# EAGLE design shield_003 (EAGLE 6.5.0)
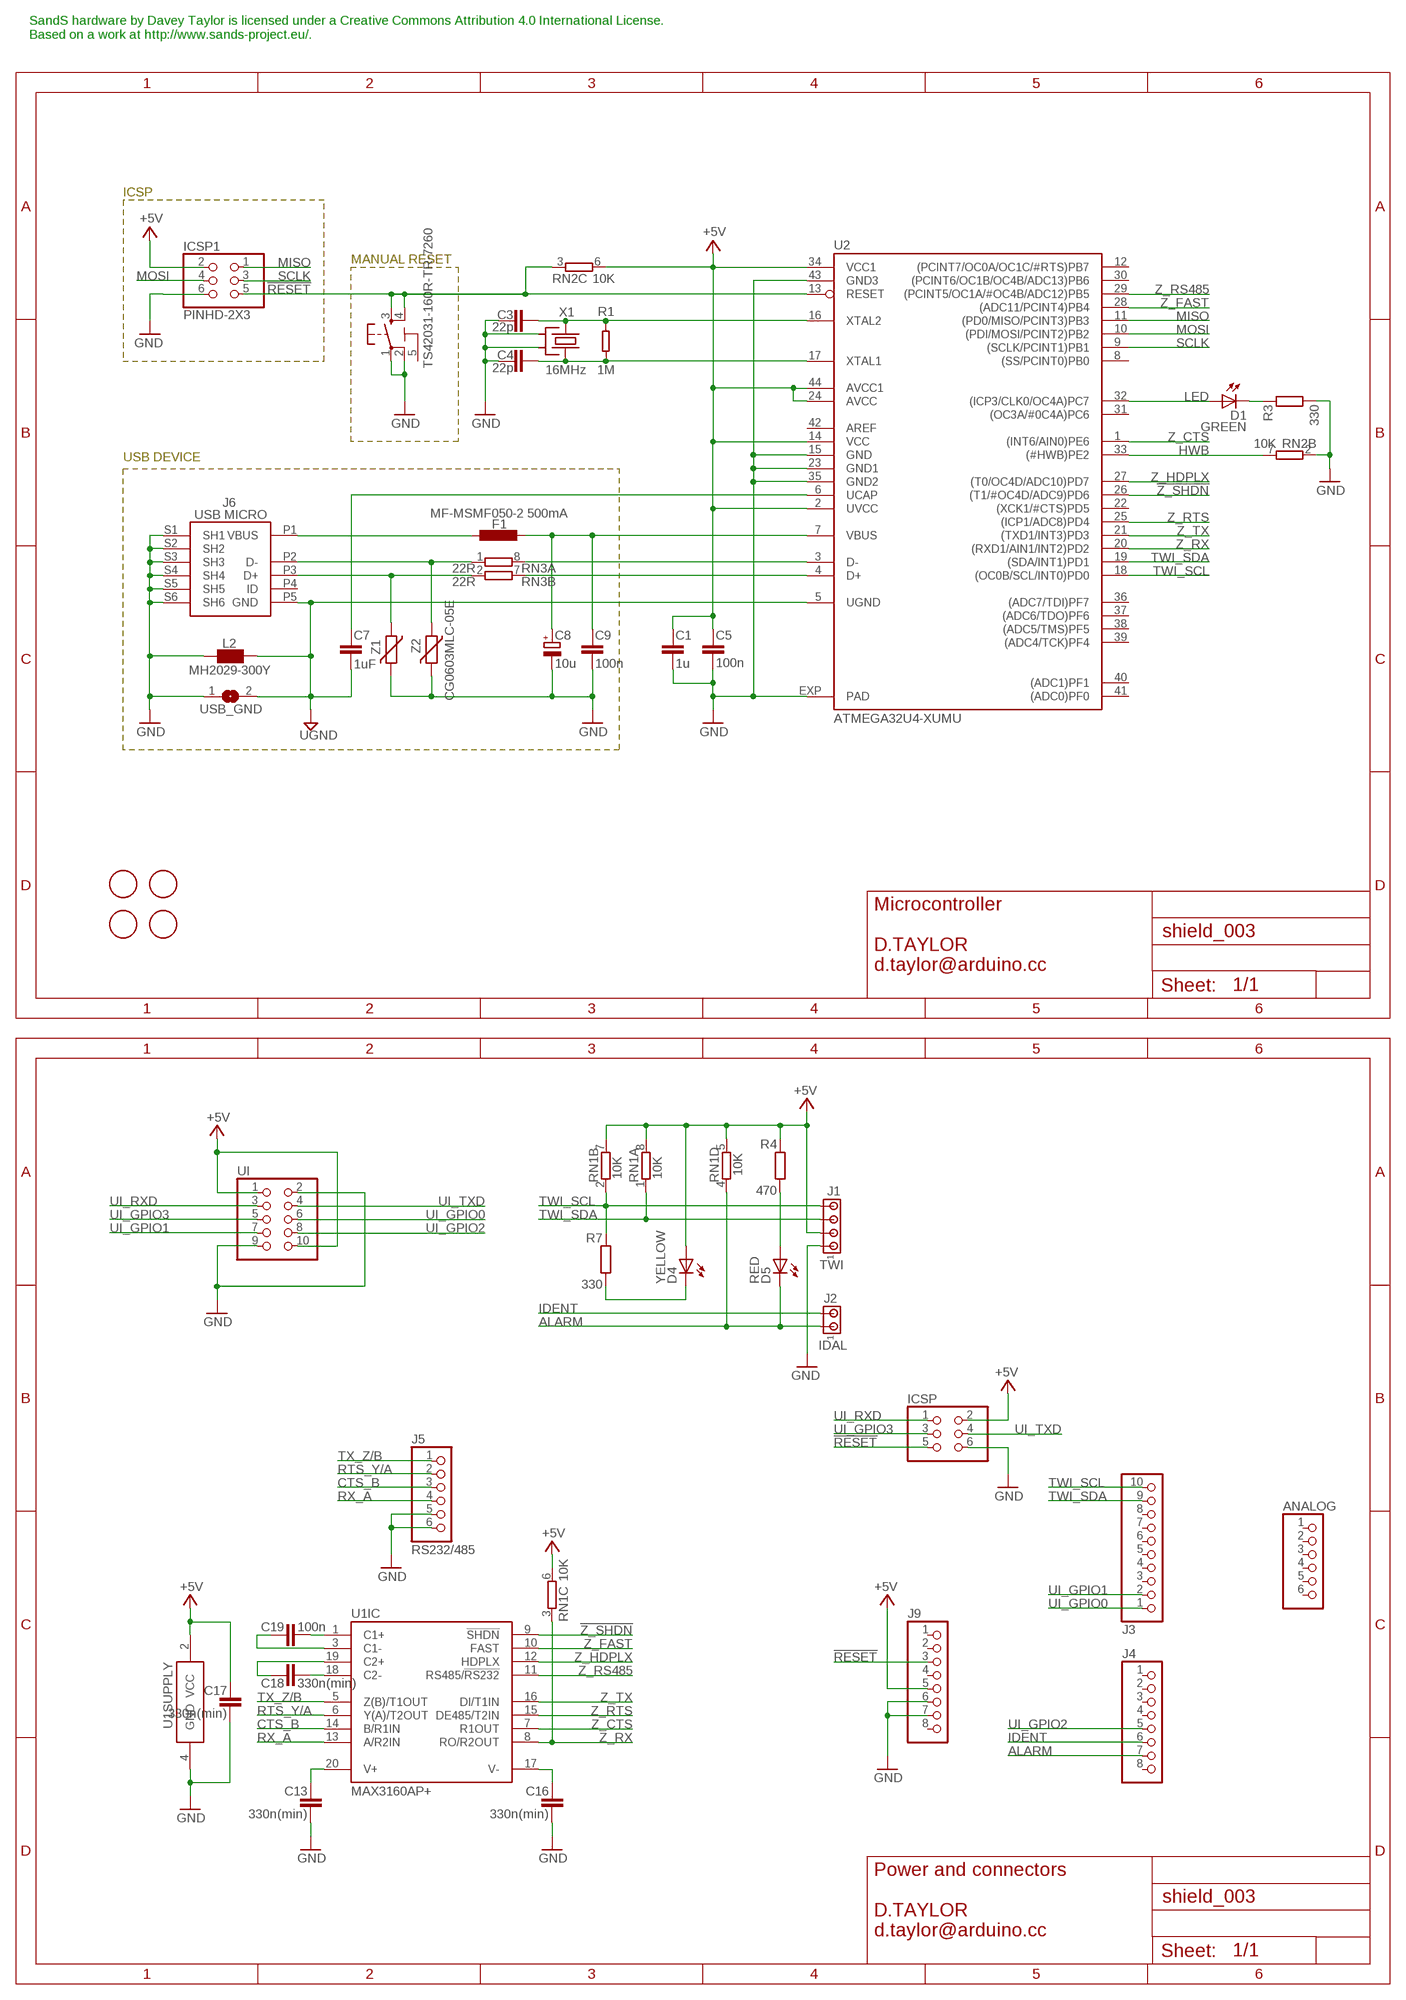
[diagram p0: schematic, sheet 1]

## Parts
ANALOG  PINHD-1X6  [1X06]
C1  1u  C-EUC0603  [C0603-ROUND]
C3  22p  C-EUC0603  [C0603-ROUND]
C4  22p  C-EUC0603  [C0603-ROUND]
C5  100n  C-EUC0603  [C0603-ROUND]
C7  1uF  C-EUC0603  [C0603-ROUND]
C8  10u  CPOL-EUSMCB  [SMC_B]
C9  100n  C-EUC0603  [C0603-ROUND]
C13  330n(min)  C-EU0603-RND  [C0603-ROUND]
C16  330n(min)  C-EU0603-RND  [C0603-ROUND]
C17  330n(min)  C-EU0603-RND  [C0603-ROUND]
C18  330n(min)  C-EU0603-RND  [C0603-ROUND]
C19  100n  C-EU0603-RND  [C0603-ROUND]
D1  GREEN  LEDCHIP-LED0805  [CHIP-LED0805]
D4  YELLOW  LEDCHIP-LED0805  [CHIP-LED0805]
D5  RED  LEDCHIP-LED0805  [CHIP-LED0805]
F1  MF-MSMF050-2 500mA  L-EUL1812  [L1812]
FID1  FIDUCIALMOUNT  [FIDUCIA-MOUNT]
FID2  FIDUCIALMOUNT  [FIDUCIA-MOUNT]
FID4  FIDUCIALMOUNT  [FIDUCIA-MOUNT]
FID5  FIDUCIALMOUNT  [FIDUCIA-MOUNT]
ICSP  PINHD-2X3  [2X03]
ICSP1  PINHD-2X3  [2X03]
J1  TWI  MTA04-100  [10X04MTA]
J2  IDAL  MTA02-100  [10X02MTA]
J3  PINHD-1X10TH  [1X10-TH]
J4  PINHD-1X8TH  [1X08-TH]
J5  RS232/485  PINHD-1X6  [1X06]
J6  USB MICRO  MYCON2_USB-MINI-B  [CON2_USB_MICRO_B_AT]
J9  PINHD-1X8TH  [1X08-TH]
L2  MH2029-300Y  WE-CBF_0805  [0805]
R1  1M  R-EU_0603-RND  [R0603-ROUND]
R3  330  R-EU_R0603  [R0603-ROUND]
R4  470  R-EU_R0603  [R0603-ROUND]
R7  330  R-EU_R0603  [R0603-ROUND]
RESET1  TS42031-160R-TR-7260  TS42  [TS42]
RN1  10K  4R-NCAT16  [CAT16]
RN2  10K  4R-NCAY16  [CAY16]
RN3  22R  4R-NCAY16  [CAY16]
U1  MAX3160AP+  [SSOP20]
U2  ATMEGA32U4-XUMU  [QFN44ML7X7]
UI  PINHD-2X5  [2X05]
USB_GND  SJ-NO  [SJ]
X1  16MHz  CRYSTAL2-KX7  [XTAL-3.2-2.5]
Z1  CG0603MLC-05E  VARISTORCN0603  [CT/CN0603]
Z2  CG0603MLC-05E  VARISTORCN0603  [CT/CN0603]

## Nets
!RESET!: ICSP1.5 ICSP.5 J9.3 RESET1.3 RESET1.4 RN2.3 U2.13(RESET)
!Z_SHDN!: U1.9(IC:!SHDN!) U2.26((T1/#OC4D/ADC9)PD6)
+5V: C1.1 C5.1 C17.1 D4.A ICSP1.2 ICSP.2 J1.2 J9.5 R4.2 RN1.5 RN1.6 RN1.7 RN1.8 RN2.6 U1.2(SUPPLY:VCC) U2.2(UVCC) U2.14(VCC) U2.24(AVCC) U2.34(VCC1) U2.44(AVCC1) UI.1 UI.10
ALARM: D5.C J2.1 J4.7 RN1.4
CTS_B: J5.3 U1.14(IC:B/R1IN)
D+: J6.P3(D+) RN3.2 Z1.1
D-: J6.P2(D-) RN3.1 Z2.1
GND: C1.2 C3.1 C4.2 C5.2 C8.- C9.2 C13.2 C16.2 C17.2 ICSP1.6 ICSP.6 J1.1 J5.5 J5.6 J6.S1(SH1) J6.S2(SH2) J6.S3(SH3) J6.S4(SH4) J6.S5(SH5) J6.S6(SH6) J9.6 J9.7 L2.2 R3.1 RESET1.1 RESET1.2 RN2.2 U1.4(SUPPLY:GND) U2.15(GND) U2.23(GND1) U2.35(GND2) U2.43(GND3) U2.EXP(PAD) UI.2 UI.9 USB_GND.1 X1.2(SH1) X1.4(SH2) Z1.2 Z2.2
HWB: RN2.7 U2.33((#HWB)PE2)
IDENT: J2.2 J4.6
LED: D1.A U2.32((ICP3/CLK0/OC4A)PC7)
MISO: ICSP1.1 U2.11((PD0/MISO/PCINT3)PB3)
MOSI: ICSP1.4 U2.10((PDI/MOSI/PCINT2)PB2)
N$2: D1.C R3.2
N$5: D5.A R4.1
N$6: C19.2 U1.1(IC:C1+)
N$7: C18.2 U1.18(IC:C2-)
N$8: C18.1 U1.19(IC:C2+)
N$9: C19.1 U1.3(IC:C1-)
N$10: C13.1 U1.20(IC:V+)
N$11: C16.1 U1.17(IC:V-)
N$14: D4.C R7.1
RTS_Y/A: J5.2 U1.6(IC:Y(A)/T2OUT)
RX_A: J5.4 U1.13(IC:A/R2IN)
SCLK: ICSP1.3 U2.9((SCLK/PCINT1)PB1)
TWI_SCL: J1.4 J3.10 R7.2 RN1.2 U2.18((OC0B/SCL/INT0)PD0)
TWI_SDA: J1.3 J3.9 RN1.1 U2.19((SDA/INT1)PD1)
TX_Z/B: J5.1 U1.5(IC:Z(B)/T1OUT)
UCAP: C7.1 U2.6(UCAP)
UGND: C7.2 J6.P5(GND) L2.1 U2.5(UGND) USB_GND.2
UI_GPIO0: J3.1 UI.6
UI_GPIO1: J3.2 UI.7
UI_GPIO2: J4.5 UI.8
UI_GPIO3: ICSP.3 UI.5
UI_RXD: ICSP.1 UI.3
UI_TXD: ICSP.4 UI.4
USB_D+: RN3.7 U2.4(D+)
USB_D-: RN3.8 U2.3(D-)
USB_VCC: C8.+ C9.1 F1.1 U2.7(VBUS)
XTAL1: C4.1 R1.1 U2.17(XTAL1) X1.3(X2)
XTAL2: C3.2 R1.2 U2.16(XTAL2) X1.1(X1)
XUSB [power usb]: F1.2 J6.P1(VBUS)
Z_CTS: U1.7(IC:R1OUT) U2.1((INT6/AIN0)PE6)
Z_FAST: U1.10(IC:FAST) U2.28((ADC11/PCINT4)PB4)
Z_HDPLX: U1.12(IC:HDPLX) U2.27((T0/OC4D/ADC10)PD7)
Z_RS485: U1.11(IC:RS485/!RS232!) U2.29((PCINT5/OC1A/#OC4B/ADC12)PB5)
Z_RTS: U1.15(IC:DE485/T2IN) U2.25((ICP1/ADC8)PD4)
Z_RX: RN1.3 U1.8(IC:RO/R2OUT) U2.20((RXD1/AIN1/INT2)PD2)
Z_TX: U1.16(IC:DI/T1IN) U2.21((TXD1/INT3)PD3)
Unconnected: ANALOG.1 ANALOG.2 ANALOG.3 ANALOG.4 ANALOG.5 ANALOG.6 J3.3 J3.4 J3.5 J3.6 J3.7 J3.8 J4.1 J4.2 J4.3 J4.4 J4.8 J6.P4(ID) J9.1 J9.2 J9.4 J9.8 RN2.1 RN2.4 RN2.5 RN2.8 RN3.3 RN3.4 RN3.5 RN3.6 U2.8((SS/PCINT0)PB0) U2.12((PCINT7/OC0A/OC1C/#RTS)PB7) U2.22((XCK1/#CTS)PD5) U2.30((PCINT6/OC1B/OC4B/ADC13)PB6) U2.31((OC3A/#0C4A)PC6) U2.36((ADC7/TDI)PF7) U2.37((ADC6/TDO)PF6) U2.38((ADC5/TMS)PF5) U2.39((ADC4/TCK)PF4) U2.40((ADC1)PF1) U2.41((ADC0)PF0)

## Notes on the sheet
- SandS hardware by Davey Taylor is licensed under a Creative Commons Attribution 4.0 International License.
  Based on a work at http://www.sands-project.eu/.
- ICSP
- MANUAL RESET
- USB DEVICE
- Microcontroller
  
  D.TAYLOR
  d.taylor@arduino.cc
- Power and connectors
  
  D.TAYLOR
  d.taylor@arduino.cc

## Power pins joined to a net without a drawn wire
5-GND: RESET1.5(5-GND)
AREF: U2.42(AREF)

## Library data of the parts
ANALOG J5 = pinhead:PINHD-1X6: PIN HEADER
C1 C3-C5 C7 C9 C13 C16-C19 = SmartPrj:C-EU: CAPACITOR, European symbol
C8 = rcl:CPOL-EU: POLARIZED CAPACITOR, European symbol
D1 D4 D5 = led:LED: LED
F1 = rcl:L-EU: INDUCTOR, European symbol
FID1 FID2 FID4 FID5 = SmartPrj:FIDUCIALMOUNT
ICSP ICSP1 = SmartPrj:PINHD-2X3: PIN HEADER
J1 = con-amp:MTA04-100: AMP connector
J2 = con-amp:MTA02-100: AMP connector
J3 = SmartPrj:PINHD-1X10: PIN HEADER
J4 J9 = SmartPrj:PINHD-1X8: PIN HEADER
J6 = d_taylor:MYCON2_USB-MINI-B
L2 = wuerth-elektronik:WE-CBF: SMD EMI Suppression Ferrite Beads
R1 = d_taylor:R-EU_: RESISTOR, European symbol
R3 R4 R7 = SmartPrj:R-EU_: RESISTOR, European symbol
RESET1 = SmartPrj:TS42: TS42 Dongnan Electronics Tact switch VDC 12V - 50mA
RN1-RN3 = resistor-dil:4R-N: Array Chip Resistor Source: RS Component / Phycomp; OC_FARNELL: unknown; OC_NEWARK: unknown
U1 = d_taylor:MAX3160*AP+
U2 = d_taylor:ATMEGA32U4-XU
UI = pinhead:PINHD-2X5: PIN HEADER
USB_GND = d_taylor:SJ?-NO: SMD solder JUMPER
X1 = d_taylor:CRYSTAL2: KX7 SMD crystal
Z1 Z2 = varistor:VARISTOR: VARISTOR

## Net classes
0 default: width 0.203 mm, drill 0.406 mm, clearance 0.203 mm
1 power: width 0.61 mm, drill 0.406 mm, clearance 0.203 mm
2 gnd: width 0.305 mm, drill 0.406 mm, clearance 0.203 mm
3 power usb: width 0.508 mm, drill 0.406 mm, clearance 0.203 mm
4 aref: width 0.203 mm, drill 0.406 mm, clearance 0.203 mm

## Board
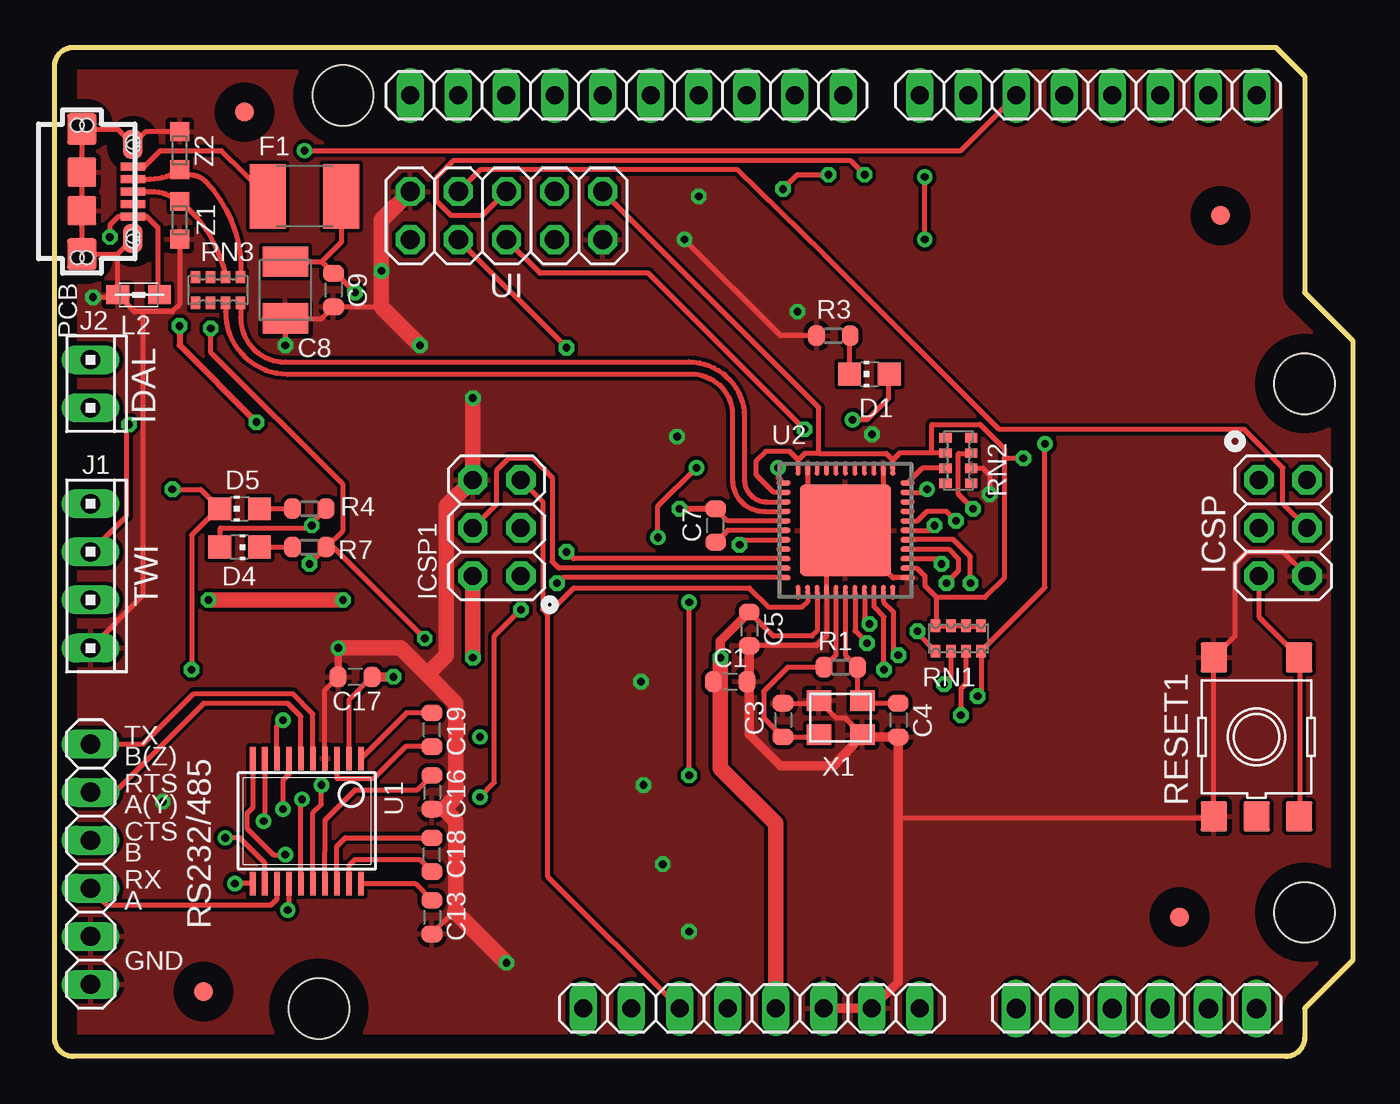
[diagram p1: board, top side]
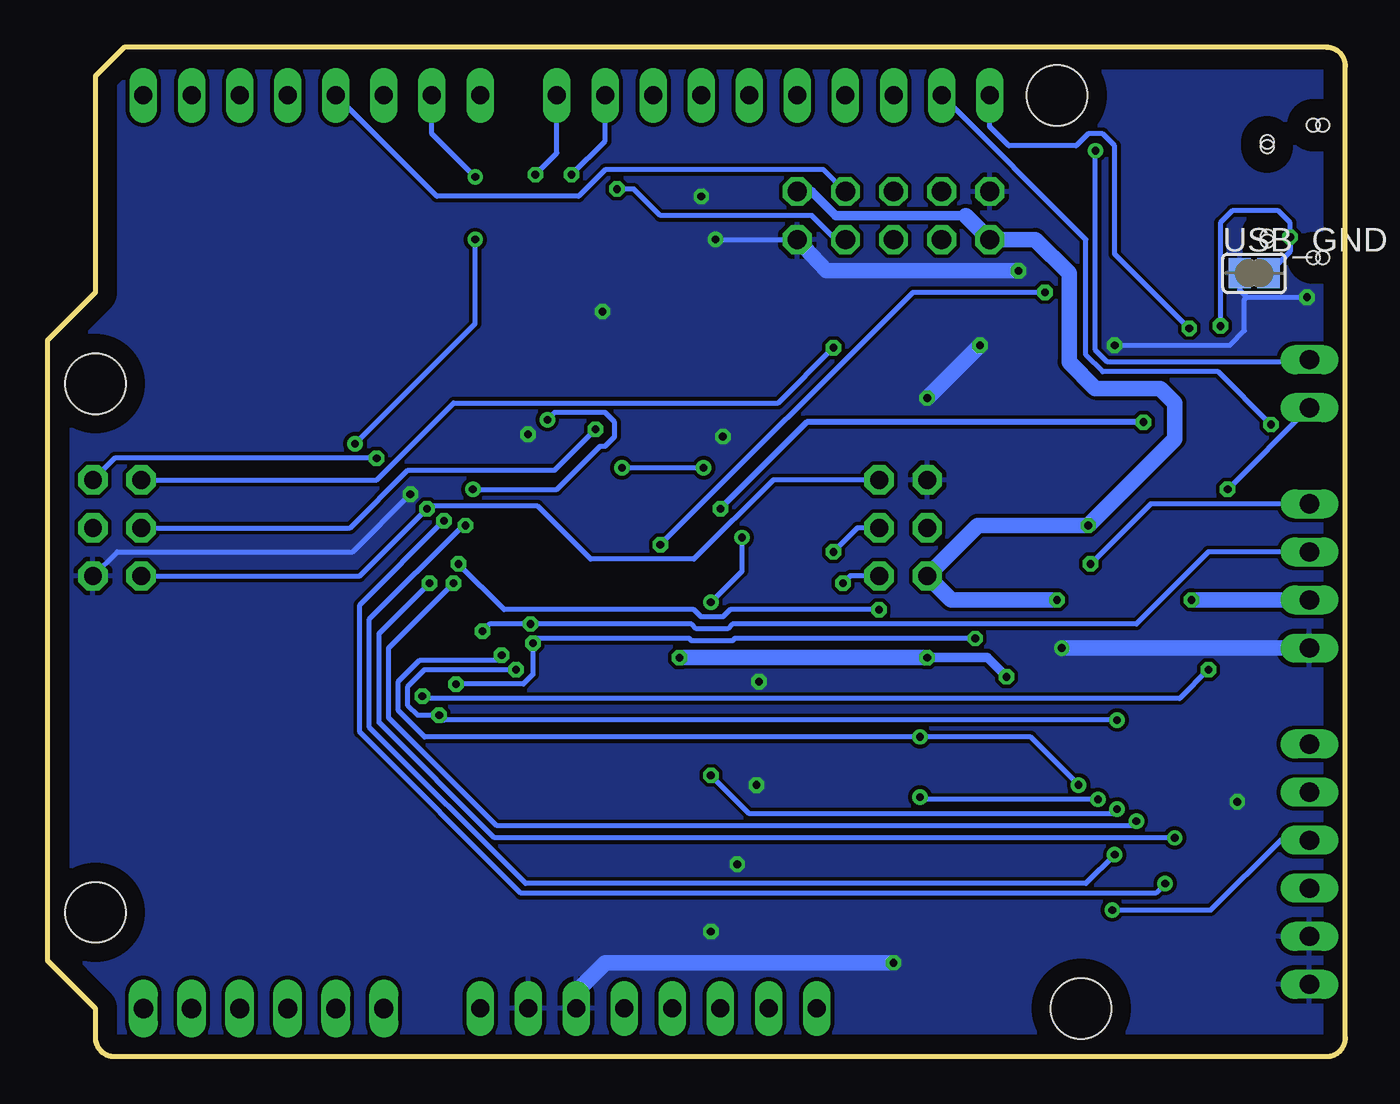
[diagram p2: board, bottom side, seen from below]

Size 68.58 x 53.34 mm. Coordinates in mm from the lower left corner, seen from the top.
Outline: 64.52,53.34 66.04,51.82 66.04,40.39 68.58,37.85 68.58,5.08 66.04,2.54 66.04,1 arc-90 65.04,0 1,0 arc-90 0,1 0,52.34 arc-90 1,53.34 64.52,53.34
Copper layers (1*16): Top 0.035mm / dielectric 1.5mm / Bottom 0.035mm
Design rules "default *": minimum track width 10mil, minimum drill 16mil, track to track 8mil, track to pad 8mil, pad to pad 8mil, via to via 8mil, smd to smd 8mil, copper to edge 40mil, drill to drill 8mil, minimum pad ring 10mil, minimum via ring 8mil, stop-mask expansion 4mil, vias tented up to drill 0mil, thermal gap 10mil
Holes 3.2 mm at 66.04,35.56 66.04,7.62 15.24,50.8 13.97,2.54

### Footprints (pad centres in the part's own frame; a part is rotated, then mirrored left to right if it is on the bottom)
1X06 = drill 1.016 long: 1 -6.35,0; 2 -3.81,0; 3 -1.27,0; 4 1.27,0; 5 3.81,0; 6 6.35,0
C0603-ROUND = smd 0.898 x 1.1: 1 -0.889,0; 2 0.889,0
SMC_B = smd 1.6 x 2.4: + -1.5,0; - 1.5,0
CHIP-LED0805 = smd 1.2 x 1.2: A 0,-1.05; C 0,1.05
L1812 = smd 1.9 x 3.4: 1 -1.95,0; 2 1.95,0
FIDUCIA-MOUNT = smd 1.016 x 1.016: P$1 0,0
2X03 = drill 0.95 pad 1.55 octagon: 1 -2.54,-1.27; 2 -2.54,1.27; 3 0,-1.27; 4 0,1.27; 5 2.54,-1.27; 6 2.54,1.27
10X04MTA = drill 1.016 long: 1 3.81,0; 2 1.27,0; 3 -1.27,0; 4 -3.81,0
10X02MTA = drill 1.016 long: 1 1.27,0; 2 -1.27,0
1X10-TH = drill 0.95 pad 1.422 long: 1 -11.43,0; 2 -8.89,0; 3 -6.35,0; 4 -3.81,0; 5 -1.27,0; 6 1.27,0; 7 3.81,0; 8 6.35,0; 9 8.89,0; 10 11.43,0
1X08-TH = drill 0.95 pad 1.422 long: 1 -8.89,0; 2 -6.35,0; 3 -3.81,0; 4 -1.27,0; 5 1.27,0; 6 3.81,0; 7 6.35,0; 8 8.89,0
CON2_USB_MICRO_B_AT = smd 0.406 x 1.346: P1 -1.321,2.692; P2 -0.66,2.692; P3 0,2.692; P4 0.66,2.692; P5 1.321,2.692 | smd 1.651 x 1.549: S1 -3.302,0; S2 3.302,0 | smd 1.524 x 1.016: S3 -2.489,2.692; S4 2.489,2.692 | smd 1.524 x 1.524: S5 -1.016,0; S6 1.016,0 | hole 0.7: -3.505,0.254; -3.505,-0.254; 3.505,0.254; 3.505,-0.254; -2.616,2.692; -2.362,2.692; 2.362,2.692; 2.616,2.692
0805 = smd 1.2 x 1: 1 -1.1,0; 2 1.1,0
R0603-ROUND = smd 0.898 x 1.1: 1 -0.889,0; 2 0.889,0
TS42 = smd 1.6 x 1.4: 1 -4.2,2.25; 2 4.2,2.25; 3 -4.2,-2.25; 4 4.2,-2.25; 5 -4.2,0
CAT16 = smd 0.5 x 0.65: 1 -1.2,-0.675; 2 -0.4,-0.675; 3 0.4,-0.675; 4 1.2,-0.675; 5 1.2,0.675; 6 0.4,0.675; 7 -0.4,0.675; 8 -1.2,0.675
CAY16 = smd 0.5 x 0.65: 1 -1.2,-0.675; 2 -0.4,-0.675; 3 0.4,-0.675; 4 1.2,-0.675; 5 1.2,0.675; 6 0.4,0.675; 7 -0.4,0.675; 8 -1.2,0.675
SSOP20 = smd 0.305 x 1.245: 1 -2.857,-3.302; 2 -2.222,-3.302; 3 -1.587,-3.302; 4 -0.952,-3.302; 5 -0.317,-3.302; 6 0.318,-3.302; 7 0.953,-3.302; 8 1.588,-3.302; 9 2.223,-3.302; 10 2.858,-3.302; 11 2.858,3.302; 12 2.223,3.302; 13 1.588,3.302; 14 0.953,3.302; 15 0.318,3.302; 16 -0.317,3.302; 17 -0.952,3.302; 18 -1.587,3.302; 19 -2.222,3.302; 20 -2.857,3.302
QFN44ML7X7 = smd 0.75 x 0.275: 1 -3.275,2.5; 2 -3.275,2; 3 -3.275,1.5; 4 -3.275,1; 5 -3.275,0.5; 6 -3.275,0; 7 -3.275,-0.5; 8 -3.275,-1; 9 -3.275,-1.5; 10 -3.275,-2; 11 -3.275,-2.5; 23 3.275,-2.5; 24 3.275,-2; 25 3.275,-1.5; 26 3.275,-1; 27 3.275,-0.5; 28 3.275,0; 29 3.275,0.5; 30 3.275,1; 31 3.275,1.5; 32 3.275,2; 33 3.275,2.5 | smd 0.275 x 0.75: 12 -2.5,-3.275; 13 -2,-3.275; 14 -1.5,-3.275; 15 -1,-3.275; 16 -0.5,-3.275; 17 0,-3.275; 18 0.5,-3.275; 19 1,-3.275; 20 1.5,-3.275; 21 2,-3.275; 22 2.5,-3.275; 34 2.5,3.275; 35 2,3.275; 36 1.5,3.275; 37 1,3.275; 38 0.5,3.275; 39 0,3.275; 40 -0.5,3.275; 41 -1,3.275; 42 -1.5,3.275; 43 -2,3.275; 44 -2.5,3.275 | smd 4.826 x 4.826: EXP 0,0
2X05 = drill 1.016 octagon: 1 -5.08,-1.27; 2 -5.08,1.27; 3 -2.54,-1.27; 4 -2.54,1.27; 5 0,-1.27; 6 0,1.27; 7 2.54,-1.27; 8 2.54,1.27; 9 5.08,-1.27; 10 5.08,1.27
SJ = smd 1.168 x 1.6: 1 -0.762,0; 2 0.762,0
XTAL-3.2-2.5 = smd 1.3 x 1.1: 1 -1.15,-0.9; 2 1.15,-0.9; 3 1.15,0.9; 4 -1.15,0.9
CT/CN0603 = smd 1 x 1: 1 -1,0; 2 1,0

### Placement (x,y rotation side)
ANALOG  57.15,2.54 0 top
C1  35.69,19.81 0 top
C3  38.48,17.78 270 top
C4  44.58,17.78 270 top
C5  36.7,22.61 270 top
C7  34.92,28.07 90 top
C8  12.19,40.51 270 top
C9  14.73,40.51 270 top
C13  19.94,7.37 270 top
C16  19.94,13.97 270 top
C17  15.88,20.07 180 top
C18  19.94,10.67 90 top
C19  19.94,17.27 90 top
D1  43.05,36.07 90 top
D4  9.78,26.92 270 top
D5  9.78,28.96 90 top
F1  13.21,45.47 180 top
FID1  10.03,49.91 0 top
FID2  7.87,3.43 0 top
FID4  61.59,44.45 0 top
FID5  59.44,7.37 0 top
ICSP  64.9,27.94 270 top
ICSP1  23.37,27.94 90 top
J1  1.91,25.4 270 top
J2  1.91,35.56 270 top
J3  30.23,50.8 180 top
J4  54.61,50.8 180 top
J5  1.91,10.16 270 top
J6  1.45,45.72 270 top
J9  36.83,2.54 0 top
L2  4.45,40.26 180 top
R1  41.53,20.57 180 top
R3  41.15,38.1 0 top
R4  13.46,28.96 0 top
R7  13.46,26.92 0 top
RESET1  63.5,16.89 90 top
RN1  47.75,22.1 0 top
RN2  47.75,31.5 90 top
RN3  8.64,40.51 180 top
U1  13.34,12.45 180 top
U2  41.78,27.81 0 top
UI  23.88,44.45 0 top
USB_GND  4.83,41.4 0 bottom
X1  41.53,17.91 0 top
Z1  6.6,44.2 270 top
Z2  6.6,47.88 90 top

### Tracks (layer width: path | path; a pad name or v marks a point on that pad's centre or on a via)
!RESET!  (via drill 0.41)
  Top 0.254: RESET1.3 65.79,12.7 65.79,21.08 RESET1.4 65.66,21.21 63.63,23.24 ICSP.5 | v48.51,28.96 47.75,29.72 47.75,31.88 48.26,31.88 RN2.3 | 26.04,23.37 27.43,24.77 36.7,24.77 37.72,23.75 39.5,23.75 39.78,24.04 U2.13 | 26.04,23.37 25.78,23.62 25.78,29.34 ICSP1.5 | J9.3 26.04,9.53 26.04,23.37
  Bottom 0.254: ICSP.5 52.07,25.4 v48.51,28.96 48.39,29.08 42.67,29.08 39.88,26.29 34.42,26.29 30.23,30.48 ICSP1.5
!Z_SHDN!  (via drill 0.41)
  Top 0.254: v47.12,25.02 47.74,25.67 47.75,25.69 47.75,26.29 47.23,26.81 U2.26 | U1.9 11.11,12.51 v11.05,12.45
  Bottom 0.254: v47.12,25.02 50.55,21.59 50.55,17.91 44.83,12.19 11.3,12.19 v11.05,12.45
+5V  (via drill 0.41)
  Top 0.254: 16.75,20.05 C17.1 15.56,18.86 U1.2 | RN2.6 46.35,31.9 | U2.14 40.28,22.5 40.01,22.23 37.97,22.23 C5.1 36.83,23.24 | 13.53,28.13 13.34,27.94 8.76,27.94 8.76,26.92 D4.A 8.64,26.92 | 13.53,28.13 R4.2 | v13.59,28.07 13.53,28.13 | RN1.5 48.9,22.73 48.26,22.73 RN1.6 RN1.7 47.24,22.73 46.61,22.73 RN1.8 46.61,22.86 46.61,24.26 | 40.39,31.88 39.62,31.88 39.28,31.54 | 46.61,24.26 49.15,24.26 50.16,25.27 50.16,31.62 | 50.16,31.62 50.16,32.13 48.9,33.4 46.35,33.4 46.35,31.9 | 50.16,31.62 v51.18,31.62 | UI.10 40.39,34.29 40.39,31.88 | 40.39,31.88 43.94,31.88 44.28,31.54 | 46.35,31.9 44.64,31.9 44.28,31.54 | U2.34 44.28,31.54 | U2.44 39.28,31.54 | U2.2 38.01,29.81 37.08,30.73 37.08,31.5 37.56,31.98 38.84,31.98 39.28,31.54 | U2.24 45.56,25.81 45.97,25.4 45.97,24.89 46.61,24.26
  Top 0.406: C1.1 35.18,19.81
  Top 0.508: v17.91,20.07 C17.1 | v35.18,21.08 35.18,21.97 C5.1
  Top 0.813: ICSP1.2 v22.1,21.08 | J9.5 38.1,12.32 35.18,15.24 35.18,19.81 v35.18,21.08 | v8.13,24.13 v15.24,24.13
  Bottom 0.254: ICSP.2 65.02,31.62 v51.18,31.62
  Bottom 0.508: v17.91,20.07 18.92,21.08 v22.1,21.08 | 20.07,44.45 26.92,44.45 28.19,45.72 UI.10
  Bottom 0.813: v8.13,24.13 J1.2 | v22.1,21.08 v35.18,21.08 | 20.07,44.45 UI.1 16.38,43.18 14.61,41.4 14.61,36.7 13.21,35.31 9.78,35.31 9.02,34.54 9.02,32.64 v13.59,28.07 19.43,28.07 ICSP1.2 20.83,24.13 v15.24,24.13
ALARM  (via drill 0.41)
  Top 0.254: v7.24,20.45 7.24,27.56 8.64,28.96 D5.C 7.71,29.97 v6.22,29.97 | 48.9,21.34 RN1.4 | RN1.4 48.95,19.23 v48.77,19.05 | RN1.4 52.32,24.8 v52.32,32.38 | v45.97,43.18 v45.97,46.48
  Bottom 0.254: v48.77,19.05 48.64,18.92 8.76,18.92 v7.24,20.45 | v6.22,29.97 J2.1 | v52.32,32.38 45.97,38.73 v45.97,43.18 | v45.97,46.48 48.26,48.77 J4.7
CTS_B  (via drill 0.41)
  Top 0.254: U1.14 12.38,7.94 v12.32,7.75
  Bottom 0.254: v12.32,7.75 7.11,7.75 3.43,11.43 J5.3
D+
  Top 0.254: J6.P3 5.08,45.72 arc-38 Z1.1 arc-42 RN3.2
D-
  Top 0.254: J6.P2 5.08,46.38 arc36 Z2.1 6.6,46.61 7.11,46.61 arc-46 8,46.23 arc-47 RN3.1
GND  (via drill 0.41)
  Top 0.254: 14.8,19.88 C17.2 14.29,19.37 U1.4 | 21.21,7.75 21.14,7.68 C13.2 | 3.33,42.42 J6.S2 J6.S6 J6.S5 J6.S1 3.33,49.02 J6.S3 4.81,48.88 Z2.2 | 3.33,42.42 J6.S4 4.19,43.18 | L2.2 3.35,42.4 3.33,42.42 | v2.03,40.13 3.22,40.13 L2.2 | Z1.2 6.6,39.75 6.22,39.37 4.7,39.37 | 4.7,39.37 4.23,39.37 L2.2 | v12.19,37.59 C8.- 14.12,39.01 C9.2 17.27,39.62 | U2.43 39.78,29.81 U2.EXP | U2.35 43.78,29.81 U2.EXP | U2.23 44.28,25.31 U2.EXP | U2.EXP 40.78,26.81 U2.15 40.78,22.24 40.26,21.72 C5.2 | C3.1 40.24,18.67 X1.4 41.28,17.91 41.78,17.91 X1.2 | 4.7,39.37 4.7,24.38 J1.1 | 61.21,12.7 61.21,21.08 RESET1.2 61.34,21.21 62.36,22.23 62.36,26.04 62.99,26.67 64.9,26.67 ICSP.6 | 61.21,12.7 61.21,12.57 44.58,12.57 | 61.21,12.7 RESET1.1 | RN2.2 49.04,31.1 49.4,30.73 v49.4,29.72 | R3.1 38.35,38.1 v33.27,43.18
  Top 0.406: v14.99,21.59 C17.2 | C1.2 36.7,19.81
  Top 0.508: 42.8,16.89 C4.2 44.58,12.57 44.58,3.94 J9.7 J9.6 | C5.2 36.7,19.81 36.7,17.02 38.35,15.37 41.17,15.37 X1.2
  Top 0.813: 20.57,13.08 21.21,12.45 21.21,7.75 | C16.2 20.57,13.08 | 20.57,13.08 21.21,13.72 21.21,18.67 19.68,20.19 | 19.68,20.19 18.29,21.59 v14.99,21.59 | UI.2 17.27,44.2 v17.27,41.53 17.27,39.62 v19.3,37.59 | v23.88,4.95 21.14,7.68 | 19.68,20.19 20.7,21.21 20.7,29.08 ICSP1.6 v22.1,34.8
  Bottom 0.254: USB_GND.1 5.59,40.51 5.21,40.13 | 5.21,40.13 v2.03,40.13 | v12.19,37.59 6.1,37.59 5.33,38.35 5.33,40.01 5.21,40.13 | v49.4,29.72 52.45,26.67 64.9,26.67 ICSP.6 | v33.27,43.18 UI.9
  Bottom 0.813: UI.9 27.43,41.53 v17.27,41.53 | v14.99,21.59 J1.1 | v23.88,4.95 39.12,4.95 40.64,3.43 J9.6 | v22.1,34.8 v19.3,37.59
  other vias: 39.24,39.37 34.04,45.47 32.89,32.77 33.53,6.6 31.11,14.35 43.18,32.89 5.71,13.46 30.99,19.81 32.13,10.16
  pour Bottom: 0.89,0.89 65.15,0.89 65.15,2.79 67.69,5.33 67.69,37.59 65.15,40.13 65.15,52.58 0.89,52.58
  pour Top: 0.89,0.89 65.15,0.89 65.15,2.79 67.69,5.33 67.69,37.59 65.15,40.13 65.15,52.58 0.89,52.58
HWB
  Top 0.254: RN2.7 45.84,31.1 U2.33
IDENT  (via drill 0.41)
  Top 0.254: v13.21,47.88 47.88,47.88 J4.6
  Bottom 0.254: J2.2 2.03,36.7 12.57,36.7 13.21,37.34 v13.21,47.88
LED  (via drill 0.41)
  Top 0.254: U2.32 45.94,29.81 v46.1,29.97 | v42.16,33.66 42.93,33.66 44.07,34.8 44.07,36.03 D1.A
  Bottom 0.254: v46.1,29.97 41.66,29.97 39.37,32.26 39.12,32.26 38.61,32.77 38.61,33.53 39.12,34.04 41.78,34.04 v42.16,33.66
MISO  (via drill 0.41)
  Top 0.254: U2.11 26.84,25.31 v26.54,25.02
  Bottom 0.254: v26.54,25.02 26.16,25.4 ICSP1.1
MOSI
  Top 0.254: ICSP1.4 23.37,29.21 23.37,30.99 24,31.62 25.27,31.62 26.29,30.61 26.29,26.16 26.64,25.81 U2.10
N$2
  Top 0.254: D1.C 42,38.07 R3.2
N$5
  Top 0.254: D5.A R4.1
N$6
  Top 0.254: C19.2 18.61,18.16 U1.1
N$7
  Top 0.254: U1.18 14.92,11.11 15.37,11.56 C18.2
N$8
  Top 0.254: U1.19 15.56,10.1 15.88,10.41 19.3,10.41 C18.1
N$9
  Top 0.254: C19.1 18.54,16.38 16.86,14.7 14.92,14.7 U1.3
N$10
  Top 0.254: U1.20 19.05,9.14 C13.1
N$11
  Top 0.254: U1.17 14.29,12.51 15.88,14.1 19.18,14.1 C16.1
N$14
  Top 0.254: D4.C R7.1
RTS_Y/A
  Top 0.254: J5.2 3.17,13.97 7.87,18.67 12.32,18.67 13.02,17.97 U1.6
RX_A
  Top 0.254: U1.13 11.75,8.32 11.43,8 2.79,8 J5.4
SCLK  (via drill 0.41)
  Top 0.254: U2.9 27.41,26.31 v27.05,26.67
  Bottom 0.254: v27.05,26.67 25.78,27.94 ICSP1.3
TWI_SCL  (via drill 0.41)
  Top 0.254: v13.46,26.04 R7.2 | v8.26,38.48 8.26,37.21 15.24,30.23 15.24,27.81 R7.2 | v42.93,21.84 42.29,22.48 42.29,24.51 U2.18 | RN1.2 47.35,20.05 v46.99,19.68 | R7.2 14.73,26.92 v19.56,22.1
  Bottom 0.254: v46.99,19.68 43.43,19.68 42.93,20.19 v42.93,21.84 42.67,22.1 34.67,22.1 34.54,21.97 32.38,21.97 32.26,22.1 v19.56,22.1 | v13.46,26.04 10.29,29.21 J1.4 | J3.10 18.8,49.15 17.78,48.13 14.22,48.13 13.59,48.77 12.83,48.77 12.19,48.13 12.19,42.42 v8.26,38.48
TWI_SDA  (via drill 0.41)
  Top 0.254: v45.59,22.48 45.59,22.35 46.48,21.46 RN1.1 | U2.19 42.8,24.51 42.8,23.11 v43.05,22.86 | v3.94,33.4 3.81,33.27 3.81,28.57 J1.3
  Bottom 0.254: v45.59,22.48 45.21,22.86 v43.05,22.86 34.54,22.86 34.29,22.61 32.64,22.61 32.38,22.86 11.05,22.86 7.24,26.67 J1.3 | J3.9 13.72,43.18 13.72,37.08 12.83,36.2 6.73,36.2 v3.94,33.4
TX_Z/B
  Top 0.254: J5.1 4.7,16.51 7.37,19.18 12.57,19.18 13.65,18.1 U1.5
UCAP
  Top 0.254: U2.6 35.56,27.81 C7.1
UGND  (via drill 0.41)
  Top 0.254: v2.92,43.31 2.92,43.94 3.38,44.4 J6.P5 4.88,44.4 5.46,43.81 5.46,40.34 L2.1 | U2.5 35.57,28.31 C7.2
  Top 0.305: v33.02,28.96 C7.2 | v10.67,33.53 6.6,37.59 v6.6,38.61
  Bottom 0.254: USB_GND.2 2.92,42.55 v2.92,43.31 2.92,44.07 3.56,44.7 5.97,44.7 6.6,44.07 v6.6,38.61
  Bottom 0.305: v33.02,28.96 28.45,33.53 v10.67,33.53
UI_GPIO0  (via drill 0.41)
  Top 0.254: UI.6 22.61,44.45 20.95,44.45 20.19,45.21 20.19,46.48 21.08,47.37 42.04,47.37 v42.8,46.61
  Bottom 0.254: v42.8,46.61 41.66,47.75 J3.1
UI_GPIO1  (via drill 0.41)
  Top 0.254: v38.48,45.85 39.24,46.61 v40.89,46.61
  Bottom 0.254: UI.7 26.92,43.18 28.19,44.45 36.2,44.45 37.59,45.85 v38.48,45.85 | v40.89,46.61 39.12,48.39 J3.2
UI_GPIO2
  Bottom 0.254: J4.5 48.01,45.47 40.51,45.47 39.12,46.86 27.56,46.86 UI.8
UI_GPIO3  (via drill 0.41)
  Top 0.254: UI.5 25.65,41.4 31.37,41.4 v39.62,33.15
  Bottom 0.254: v39.62,33.15 41.78,30.99 49.53,30.99 52.58,27.94 ICSP.3
UI_RXD  (via drill 0.41)
  Top 0.254: v27.05,37.47 UI.3
  Bottom 0.254: v27.05,37.47 29.97,34.54 47.12,34.54 51.18,30.48 ICSP.1
UI_TXD
  Top 0.254: UI.4 22.48,46.86 36.07,46.86 40.64,42.42 49.91,33.15 62.87,33.15 64.9,31.11 64.9,29.21 ICSP.4
USB_D+
  Top 0.254: RN3.7 9.04,39.35 arc90 12.32,36.07 33.66,36.07 arc-90 35.81,33.91 35.81,30.48 arc90 37.48,28.81 U2.4
USB_D-
  Top 0.254: RN3.8 9.84,39.06 arc90 12.19,36.7 33.53,36.7 arc-90 36.45,33.78 36.45,30.48 arc90 37.62,29.31 U2.3
USB_VCC  (via drill 0.41)
  Top 0.254: C8.+ 14.12,42.01 | 14.12,42.01 C9.1 14.73,41.53 v15.88,40.39 | F1.1 15.16,43.05 14.12,42.01 | v36.2,27.05 36.2,27.3 38.48,27.3 U2.7
  Bottom 0.254: v36.2,27.05 22.86,40.39 v15.88,40.39
XTAL1
  Top 0.254: U2.17 41.78,21.21 R1.1 42.42,19.07 X1.3 42.82,18.67 C4.1
XTAL2
  Top 0.254: U2.16 41.28,21.22 R1.2 | R1.2 40.39,20.57 | X1.1 40.26,16.89 C3.2 37.47,17.91 37.47,19.3 38.73,20.57 R1.2
XUSB
  Top 0.254: J6.P1 4.75,47.04 5.59,47.88 8.81,47.88 F1.2
Z_CTS  (via drill 0.41)
  Top 0.254: U1.7 12.38,14.92 12.06,14.61 v12.06,13.08 | v33.53,14.86 v33.53,24 | v31.88,27.43 31.88,29.08 v33.91,31.11 | v38.23,31.11 38.23,30.59 U2.1
  Bottom 0.254: v33.53,14.86 31.5,12.83 12.32,12.83 v12.06,13.08 | v33.53,24 31.88,25.65 v31.88,27.43 | v33.91,31.11 v38.23,31.11
Z_FAST  (via drill 0.41)
  Top 0.254: U2.28 46.23,27.81 v46.48,28.07 | U1.10 10.48,13.14 10.16,12.83 10.16,12.06 11.56,10.67 v12.19,10.67
  Bottom 0.254: v12.19,10.67 13.72,9.14 43.31,9.14 51.56,17.4 51.56,23.11 46.61,28.07 v46.48,28.07
Z_HDPLX  (via drill 0.41)
  Top 0.254: 45.47,27.31 U2.27 47.49,27.31 48.39,26.42 v48.39,25.02 | U1.12 11.11,10.22 9.78,11.56 v9.02,11.56
  Bottom 0.254: v9.02,11.56 44.96,11.56 51.05,17.65 51.05,22.35 v48.39,25.02
Z_RS485  (via drill 0.41)
  Top 0.254: U2.29 45.59,28.31 46.1,28.83 47.12,28.83 v47.62,28.32 | U1.11 v9.53,9.14
  Bottom 0.254: v9.53,9.14 10.03,8.64 43.56,8.64 52.07,17.14 52.07,23.88 v47.62,28.32
Z_RTS  (via drill 0.41)
  Top 0.254: v24.64,23.62 23.24,22.23 23.24,14.48 v22.48,13.72 | U2.25 46.59,26.31 v46.86,26.04 | U1.15 13.02,13.53 v13.08,13.59
  Bottom 0.254: v13.08,13.59 22.35,13.59 v22.48,13.72 | v46.86,26.04 44.45,23.62 34.42,23.62 34.04,23.24 32.89,23.24 32.51,23.62 v24.64,23.62
Z_RX  (via drill 0.41)
  Top 0.254: v43.81,20.45 43.81,23.24 43.28,23.77 U2.20 | RN1.3 48.15,19.7 47.88,19.43 v47.88,18.03 | U1.8 11.75,17.46 v12.06,17.78
  Bottom 0.254: v12.06,17.78 47.62,17.78 v47.88,18.03 49.02,18.03 49.53,18.54 49.53,19.56 48.64,20.45 v43.81,20.45
Z_TX  (via drill 0.41)
  Top 0.254: v44.58,21.21 44.32,21.46 44.32,23.5 43.78,24.04 U2.21 | U1.16 13.65,12.89 14.1,13.34 v14.1,14.35
  Bottom 0.254: v14.1,14.35 16.64,16.89 v22.48,16.89 48.64,16.89 50.04,18.29 50.04,19.81 48.9,20.95 44.83,20.95 v44.58,21.21

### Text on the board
tPlace: TX / B(Z) | RTS / A(Y) | CTS / B | RX / A | GND
tSilk: ALARM | ACT | ACTIVITY | COMM | RESET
